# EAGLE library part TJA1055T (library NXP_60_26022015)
Enhanced fault-tolerant CAN transceiver The TJA1055 is the interface between the protocol controller and the physical bus wires in a Controller Area Network (CAN). It is primarily intended for low-speed applications up to 125 kBd in passenger cars. The device provides differential receive and transmit capability but will switch to single-wire transmitter and/or receiver in error conditions. The TJA1055 is the enhanced version of the TJA1054 and TJA1054A. TJA1055 has the same functionality but in addition offering a number of improvements. The most important improvements of the TJA1055 with respect to the TJA1054 and TJA1054A are: Improved ElectroStatic Discharge (ESD) performance Lower current consumption in sleep mode Wake-up signalling on RXD and ERR without VCC active 3 V interfacing with microcontroller possible with TJA1055T/3 AAL Eindhoven MK
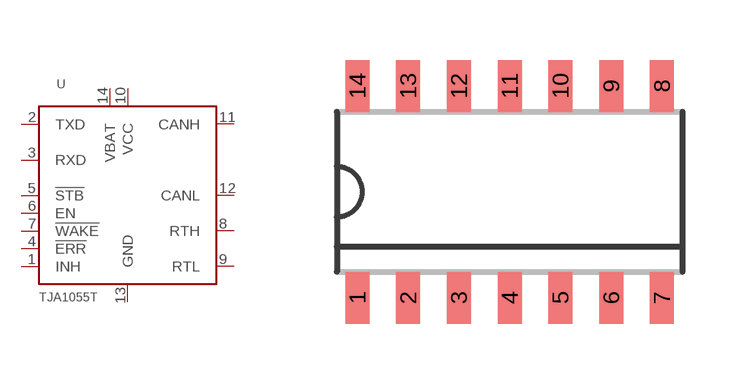
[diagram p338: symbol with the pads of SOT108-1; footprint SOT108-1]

Designator prefix U

## TJA1055T  [SOT108-1]
1  INH  in
2  TXD  out
3  RXD
4  !ERR  out
5  !STB  in
6  EN  in
7  !WAKE  in
8  RTH  pas
9  RTL  pas
10  VCC  pwr
11  CANH
12  CANL
13  GND  pwr
14  VBAT  pwr

## Footprint SOT108-1 (pad centres in mm)
SOT108-1 SO14: plastic small outline package; 14 leads; body width 3.9 mm; body thickness 1.47 mm JEDEC: MS-012 IEC: --
smd 0.6 x 1.3: 1 -3.81,-2.65; 2 -2.54,-2.65; 3 -1.27,-2.65; 4 0,-2.65; 5 1.27,-2.65; 6 2.54,-2.65; 7 3.81,-2.65; 8 3.81,2.65; 9 2.54,2.65; 10 1.27,2.65; 11 0,2.65; 12 -1.27,2.65; 13 -2.54,2.65; 14 -3.81,2.65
